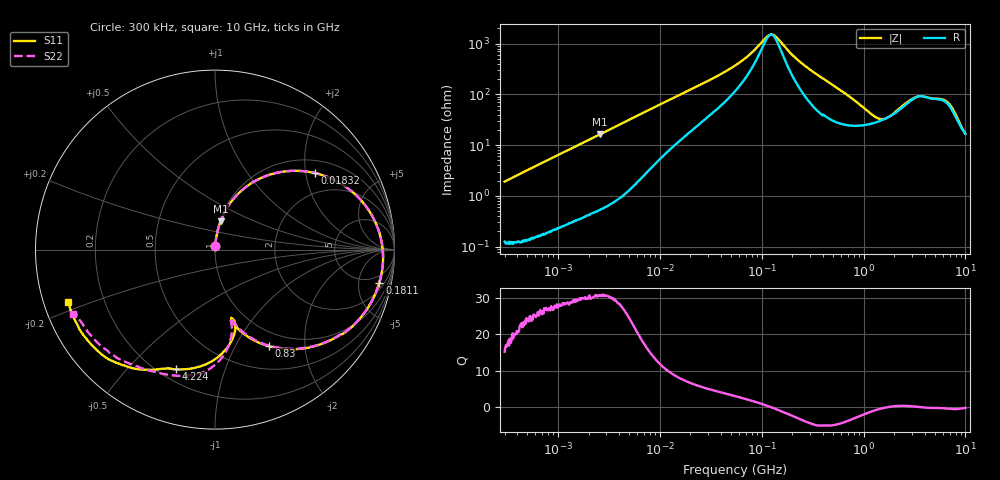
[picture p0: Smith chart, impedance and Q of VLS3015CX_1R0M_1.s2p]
! S-Parameter Data Generated by TDK Corporation
! Copyright(C) 2019 TDK Corporation.
! All Rights Reserved.
! TDK P/N: VLS3015CX-1R0M-1 (Inductor)
! Property: L=1uH at 1MHz
! Size(LxWxT): 3x3x1.5mm
! Model Type: s2p (Touchstone File Format Version 1.0)
! Frequency: DC=Yes Start=0.3MHz Stop=10000MHz 802points Log-sweep
! Model Generated on Sep. 23, 2019
! Port Assignments:
!  1 ---@@@--- 2
! Applicable Conditions:
!  Temperature = 25 degC
!  DC Bias Current = 0 A
!  Small Signal Operation
! Terms and conditions regarding TDK Simulation Models
! (1)This simulation model is being provided solely for informational purposes. Please refer to the specifications of the products in terms of detailed characteristics of such products.
! (2)In no event shall TDK Corporation of any of its subsidiaries be liable for any loss or damage arising, directly or indirectly,
!  From any information contained in this simulation model, including, but not limited to loss or damages arising from any inaccuracies, omissions or errors in connection with such information.
! (3)Any and all copyrights on this simulation model are owned by TDK Corporation.
!  Duplication or redistribution of this simulation model without prior written permission from TDK Corporation is prohibited.
! (4)This simulation model is subject to any modification or change without any prior notice.
! (5)Neither TDK Corporation nor any of its subsidiaries shall make any warranty, express or implied,
!  Including but not limited to the correctness, implied warranties of merchantability and fitness for a particular purpose with respect to this simulation models.
! (6)The use of this simulation model shall be deemed to have consented to the terms and conditions hereof.
# Hz S MA R 50
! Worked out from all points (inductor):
!   801 points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, 300 kHz to 10 GHz, reference 50 ohm
!   read as one part in series: L = 1.02 uH near 318.3 kHz
!   highest Q = 30.7 at 2.599 MHz (marker M1), where L = 1 uH
!   self-resonance near 123.7 MHz
!   S11 on the Smith chart (normalised r, x): 300 kHz: 1.00, +0.04; 18.32 MHz: 1.34, +2.26; 181.1 MHz: 3.13, -9.02; 830 MHz: 0.80, -1.38; 4.224 GHz: 0.26, -0.69; 10 GHz: 0.07, -0.17
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300000  0.01896 85.1  0.9984 -1.1  0.9987 -1.1  0.01878 85.0
1713600  0.107 81.9  0.9906 -6.2  0.9907 -6.2  0.1069 81.9
2598892  0.16 78.9  0.9819 -9.3  0.9818 -9.3  0.16 78.8
5292453  0.3116 69.3  0.9369 -18.3  0.9369 -18.3  0.3115 69.3
9671944  0.5009 55.1  0.8256 -30.2  0.8258 -30.2  0.501 55.1
1.831589e7  0.702 37.4  0.6204 -44.5  0.6204 -44.5  0.7019 37.4
5.477226e7  0.8966 11.9  0.2438 -59.9  0.2438 -59.9  0.8965 11.9
1.210198e8  0.9378 -3.0  0.06251 -8.5  0.06255 -8.5  0.9377 -2.9
1.372768e8  0.9387 -5.4  0.06778 20.6  0.06778 20.6  0.9386 -5.4
1.810762e8  0.9343 -11.3  0.126 50.6  0.126 50.6  0.934 -11.2
3.126428e8  0.8929 -25.8  0.3014 52.3  0.3014 52.3  0.8927 -25.6
5.285151e8  0.7767 -43.7  0.4977 35.8  0.4977 35.7  0.7765 -43.4
8.299813e8  0.6147 -60.9  0.6412 14.3  0.6412 14.3  0.6143 -60.6
1.228555e9  0.4704 -73.0  0.6971 -7.9  0.697 -7.9  0.4703 -72.3
1.767019e9  0.3924 -76.8  0.6663 -31.6  0.6662 -31.5  0.3991 -76.3
2.172958e9  0.4215 -74.8  0.5971 -46.2  0.5974 -46.1  0.4131 -77.3
2.659614e9  0.5115 -79.3  0.4945 -58.8  0.4946 -58.8  0.4931 -79.4
3.387826e9  0.641 -94.4  0.3633 -66.6  0.3634 -66.6  0.6355 -89.3
4.22443e9  0.7019 -108.2  0.3084 -67.2  0.3087 -67.2  0.7184 -102.2
6.899057e9  0.8289 -129.9  0.2193 -80.0  0.2189 -80.0  0.8113 -131.3
8.546531e9  0.8742 -146.8  0.2042 -85.8  0.204 -85.8  0.8464 -150.1
1e10  0.8674 -160.4  0.1957 -92.0  0.1958 -91.9  0.8667 -155.7
